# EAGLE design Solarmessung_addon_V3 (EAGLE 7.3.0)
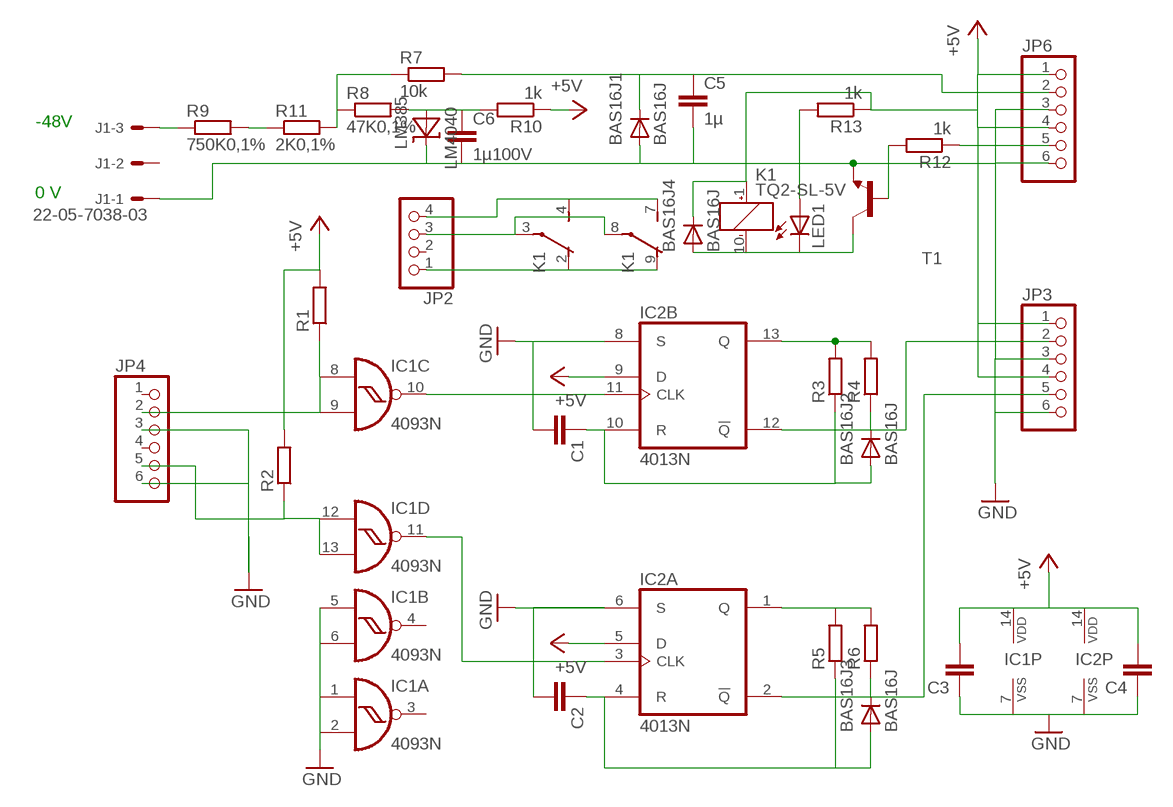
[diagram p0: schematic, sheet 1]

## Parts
BAS16J1  BAS16J  [SOD323-W]
BAS16J2  BAS16J  [SOD323-W]
BAS16J3  BAS16J  [SOD323-W]
BAS16J4  BAS16J  [SOD323-W]
C1  C-EUC1206  [C1206]
C2  C-EUC1206  [C1206]
C3  C-EUC1206  [C1206]
C4  C-EUC1206  [C1206]
C5  1µ  C-EUC0805  [C0805]
C6  1µ100V  C-EUC1206  [C1206]
IC1  4093N  [DIL14]
IC2  4013N  [DIL14]
J1  22-05-7038-03  [7395-03]
JP2  PINHD-1X4  [1X04]
JP3  PINHD-1X6  [1X06]
JP4  PINHD-1X6  [1X06]
JP6  PINHD-1X6  [1X06]
K1  TQ2-SL-5V  [TQ-SL]
LED1  LED3MM  [LED3MM]
LM4040  LM385  [TO-92]
R1  R-EU_R1206  [R1206]
R2  R-EU_R1206  [R1206]
R3  R-EU_R0603  [R0603]
R4  R-EU_R0603  [R0603]
R5  R-EU_R0603  [R0603]
R6  R-EU_R0603  [R0603]
R7  10k  R-EU_M1206  [M1206]
R8  47K0,1%  R-EU_M1206  [M1206]
R9  750K0,1%  R-EU_M1206  [M1206]
R10  1k  R-EU_M1206  [M1206]
R11  2K0,1%  R-EU_M1206  [M1206]
R12  1k  R-EU_R0603  [R0603]
R13  1k  R-EU_R0603  [R0603]
T1  -NPN-SOT23-EBC  [SOT23-EBC]

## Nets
+5V: BAS16J4.C C3.2 C4.2 IC1.14(P:VDD) IC2.5(A:D) IC2.9(B:D) IC2.14(P:VDD) JP3.1 JP3.4 JP6.1 JP6.4 K1.1(_:+) R1.2 R2.2 R10.1 R13.1
GND: BAS16J1.A C1.2 C2.2 C3.1 C4.1 C5.2 C6.2 IC1.1(A:I0) IC1.2(A:I1) IC1.5(B:I0) IC1.6(B:I1) IC1.7(P:VSS) IC2.6(A:S) IC2.7(P:VSS) IC2.8(B:S) J1.1 JP3.3 JP3.6 JP4.3 JP4.6 JP6.3 JP6.6 LM4040.- T1.E
N$1: IC1.8(C:I0) IC1.9(C:I1) JP4.2 R1.1
N$2: IC1.12(D:I0) IC1.13(D:I1) JP4.5 R2.1
N$3: C6.1 LM4040.+ R8.2 R10.2
N$4: IC1.10(C:O) IC2.11(B:CLK)
N$5: BAS16J2.C R4.1
N$6: BAS16J2.A C1.1 IC2.10(B:R) R3.1
N$7: IC2.13(B:Q) R3.2 R4.2
N$8: IC1.11(D:O) IC2.3(A:CLK)
N$9: BAS16J3.C R6.1
N$10: BAS16J3.A C2.1 IC2.4(A:R) R5.1
N$11: IC2.1(A:Q) R5.2 R6.2
N$12: J1.3 R9.1
N$13: R7.1 R8.1 R11.2
N$14: BAS16J1.C C5.1 JP6.2 R7.2
N$15: R9.2 R11.1
N$16: R12.2 T1.B
N$17: JP6.5 R12.1
N$18: BAS16J4.A K1.10(_:-) LED1.K(C) T1.C
N$19: JP2.4 K1.4(1:S) K1.7(2:S)
N$20: JP2.3 K1.3(1:P) K1.8(2:P)
N$21: JP2.1 K1.2(1:O) K1.9(2:O)
N$22: IC2.12(B:!Q) JP3.2
N$23: LED1.A R13.2
N$24: IC2.2(A:!Q) JP3.5
Unconnected: IC1.3(A:O) IC1.4(B:O) J1.2 JP2.2 JP4.1 JP4.4

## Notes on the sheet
- -48V
- 0 V

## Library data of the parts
BAS16J1-BAS16J4 = diode:BAS16J
C1-C6 = rcl:C-EU: CAPACITOR, European symbol
IC1 = 40xx:4093: Quad 2-input NAND schmitt trigger
IC2 = 40xx:4013: Dual D FLIP FLOP, set/reset
J1 = con-molex:22-?-03: CONNECTOR wire to board 2.54 mm (.1 inch) pitch header
JP2 = pinhead:PINHD-1X4: PIN HEADER
JP3 JP4 JP6 = pinhead:PINHD-1X6: PIN HEADER
K1 = relay:TQ2?*: LOW PROFILE 2 FORM C RELAY NAiS Source: http://www.mew-europe.com/.. en_ds_61020_0001.pdf Source: http://www.mew-europe.com/.. en_ds_61020_0004.pdf
LED1 = led:LED: LED
LM4040 = lm385:LM385: LM385
R1-R13 = rcl:R-EU_: RESISTOR, European symbol
T1 = transistor:*-NPN-: NPN Transistror BF959 corrected 2008.03.06

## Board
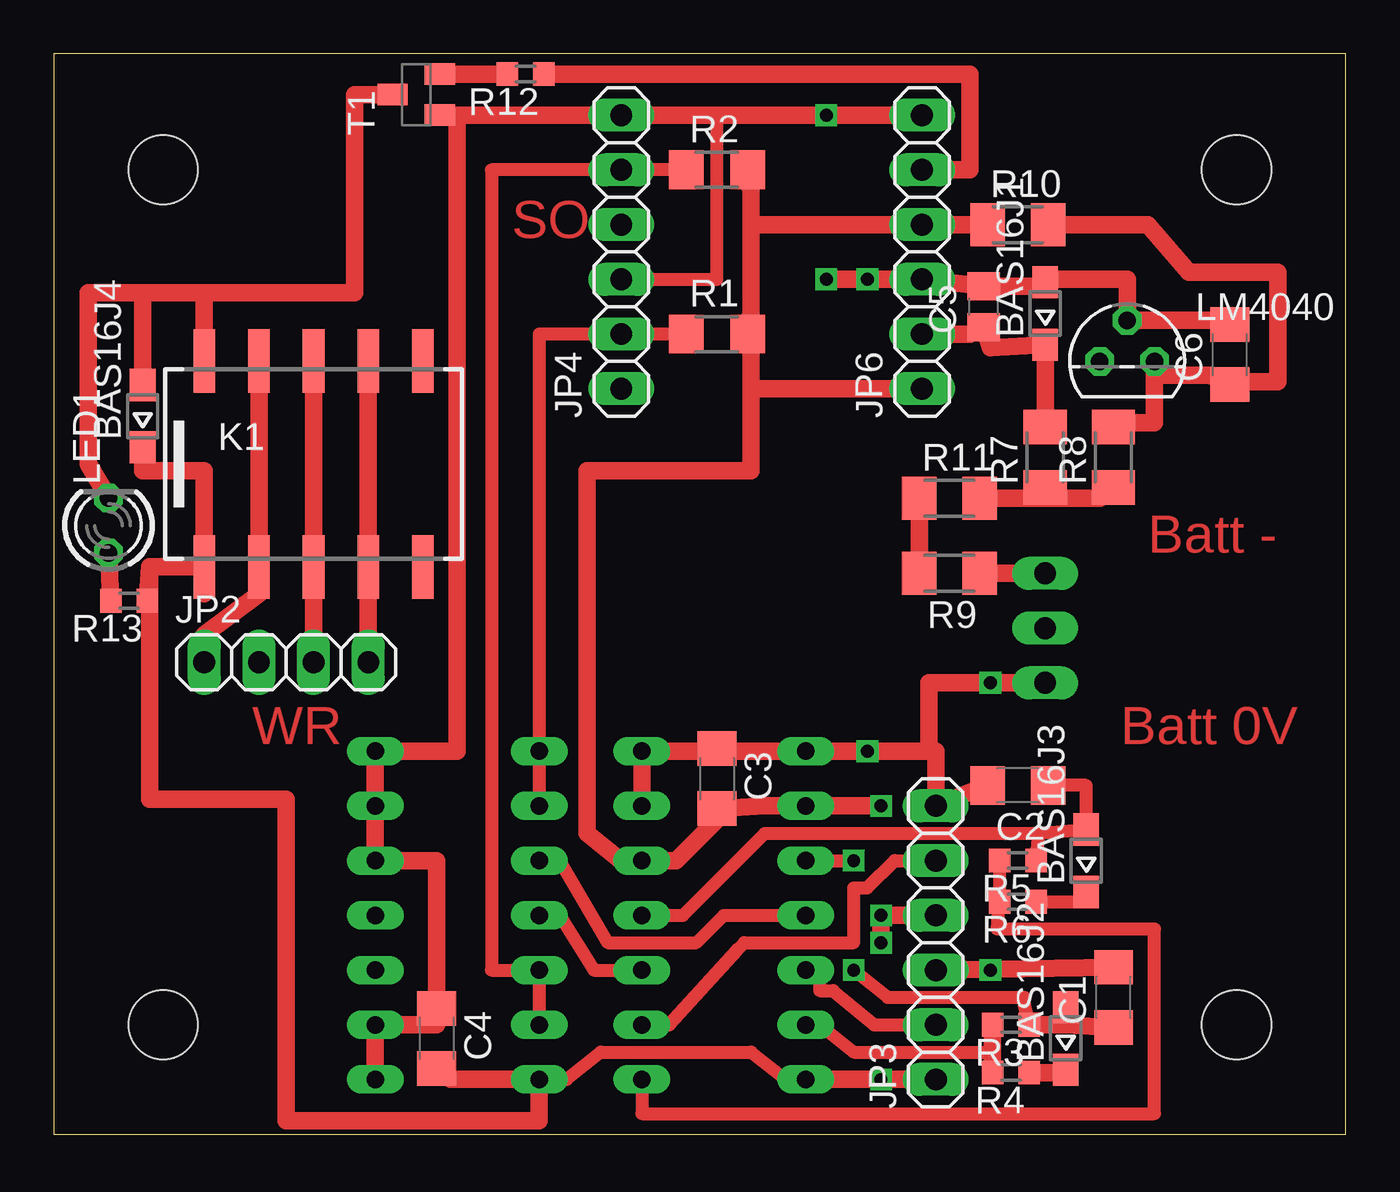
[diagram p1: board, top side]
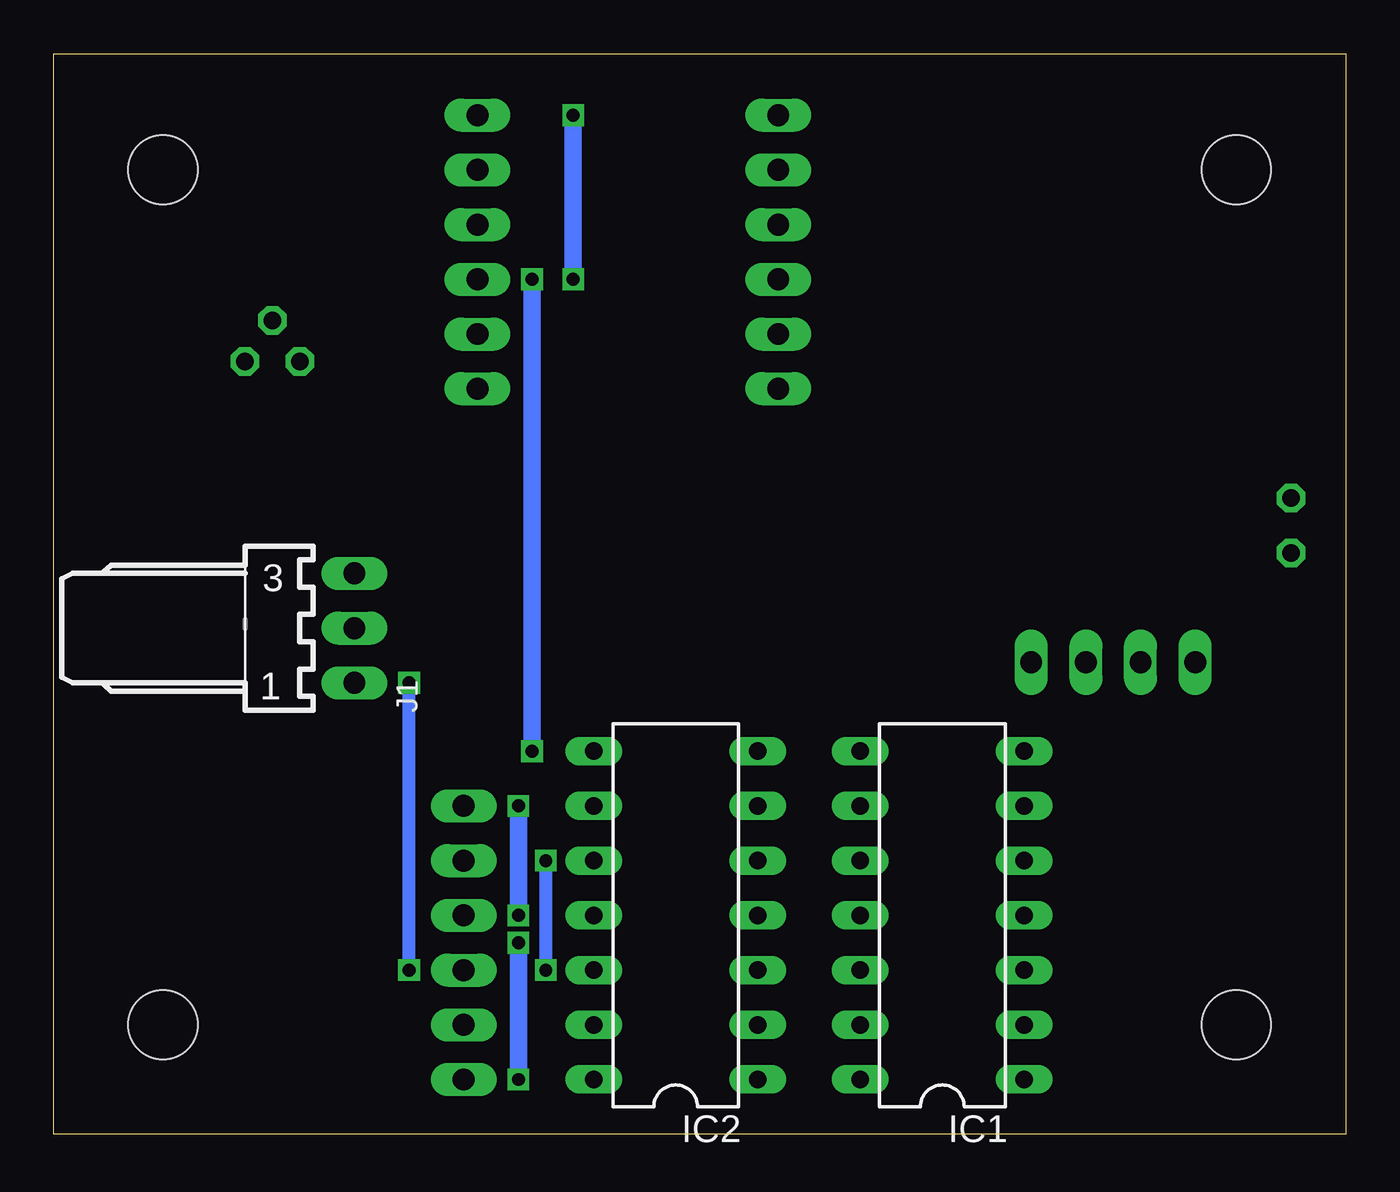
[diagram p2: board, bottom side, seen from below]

Size 59.99 x 50.16 mm. Coordinates in mm from the lower left corner, seen from the top.
Outline: 0,0 59.99,0 59.99,50.16 0,50.16 0,0
Copper layers (1*16): Top 0.035mm / dielectric 1.5mm / Bottom 0.035mm
Design rules "default": minimum track width 10mil, minimum drill 24mil, track to track 8mil, track to pad 8mil, pad to pad 8mil, via to via 8mil, smd to smd 8mil, copper to edge 40mil, drill to drill 8mil, minimum pad ring 10mil, minimum via ring 8mil, stop-mask expansion 4mil, vias tented up to drill 0mil, thermal gap 10mil
Holes 3.2 mm at 5.08,5.08 54.93,5.08 5.08,44.77 54.93,44.77

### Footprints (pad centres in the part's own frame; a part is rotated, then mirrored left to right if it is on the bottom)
SOD323-W = smd 1.5 x 1.2: A 1.45,0; C -1.45,0
C1206 = smd 1.6 x 1.8: 1 -1.4,0; 2 1.4,0
C0805 = smd 1.3 x 1.5: 1 -0.95,0; 2 0.95,0
DIL14 = drill 0.813 long: 1 -7.62,-3.81; 2 -5.08,-3.81; 3 -2.54,-3.81; 4 0,-3.81; 5 2.54,-3.81; 6 5.08,-3.81; 7 7.62,-3.81; 8 7.62,3.81; 9 5.08,3.81; 10 2.54,3.81; 11 0,3.81; 12 -2.54,3.81; 13 -5.08,3.81; 14 -7.62,3.81
7395-03 = drill 1.016 long: 1 2.54,0; 2 0,0; 3 -2.54,0
1X04 = drill 1.016 long: 1 -3.81,0; 2 -1.27,0; 3 1.27,0; 4 3.81,0
1X06 = drill 1.016 long: 1 -6.35,0; 2 -3.81,0; 3 -1.27,0; 4 1.27,0; 5 3.81,0; 6 6.35,0
TQ-SL = smd 1 x 2.94: 1 -5.08,-4.78; 2 -2.54,-4.78; 3 0,-4.78; 4 2.54,-4.78; 5 5.08,-4.78; 6 5.08,4.78; 7 2.54,4.78; 8 0,4.78; 9 -2.54,4.78; 10 -5.08,4.78
LED3MM = drill 0.813 octagon: A -1.27,0; K 1.27,0
TO-92 = drill 0.813 octagon: + 1.27,0; - 0,1.905; NC -1.27,0
R1206 = smd 1.6 x 1.803: 1 -1.422,0; 2 1.422,0
R0603 = smd 1 x 1.1: 1 -0.85,0; 2 0.85,0
M1206 = smd 1.6 x 2: 1 -1.4,0; 2 1.4,0
SOT23-EBC = smd 1 x 1.4: B 0.95,-1.1; C 0,1.1; E -0.95,-1.1

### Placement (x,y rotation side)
BAS16J1  46.04,38.1 90 top
BAS16J2  46.99,4.45 90 top
BAS16J3  47.94,12.7 90 top
BAS16J4  4.13,33.34 90 top
C1  49.21,6.35 90 top
C2  44.77,16.19 180 top
C3  30.8,16.51 270 top
C4  17.78,4.45 270 top
C5  43.18,38.42 90 top
C6  54.61,36.2 90 top
IC1  18.73,10.16 90 bottom
IC2  31.11,10.16 90 bottom
J1  46.04,23.5 270 bottom
JP2  10.79,21.91 0 top
JP3  40.96,8.89 90 top
JP4  26.35,40.96 90 top
JP6  40.32,40.96 90 top
K1  12.06,31.11 0 top
LED1  2.54,28.26 90 top
LM4040  49.85,35.88 0 top
R1  30.8,37.15 0 top
R2  30.8,44.77 0 top
R3  44.45,5.08 180 top
R4  44.45,2.86 180 top
R5  44.77,12.7 180 top
R6  44.77,10.79 180 top
R7  46.04,31.43 90 top
R8  49.21,31.43 90 top
R9  41.59,26.04 180 top
R10  44.77,42.23 0 top
R11  41.59,29.53 0 top
R12  21.91,49.21 180 top
R13  3.49,24.77 180 top
T1  16.83,48.26 90 top

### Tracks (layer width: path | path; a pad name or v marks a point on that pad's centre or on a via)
+5V  (via drill 0.6)
  Top 0.61: IC1.14 23.81,2.54 25.4,3.81 32.38,3.81 33.97,2.54 IC2.14 | 34.29,15.24 IC2.9
  Top 0.813: R10.1 JP6.4 32.38,42.23 | IC2.14 v38.42,2.54 JP3.1 | BAS16J4.C 4.13,30.8 6.99,30.8 6.99,26.35 | 6.99,25.08 K1.1 6.99,26.35 | 4.45,26.35 R13.1 | 6.99,26.35 4.45,26.35 | 4.45,26.35 4.45,15.56 10.79,15.56 10.79,0.64 22.54,0.64 IC1.14 18.41,2.54 C4.2 | v38.42,8.89 v38.42,10.16 JP3.4 | v38.42,15.24 34.29,15.24 33.02,15.24 C3.2 30.8,14.61 28.89,12.7 IC2.5 26.35,12.7 24.77,13.97 24.77,30.8 32.38,30.8 32.38,34.61 | 32.38,42.23 32.38,43.81 R2.2 | 32.38,42.23 32.38,38.1 R1.2 32.38,36.51 32.38,34.61 | JP6.1 32.38,34.61
  Bottom 0.813: v38.42,8.89 v38.42,2.54 | v38.42,10.16 v38.42,15.24
GND  (via drill 0.6)
  Top 0.61: 43.18,16.19 C2.2 | 30.8,47.31 JP4.6 19.05,47.31 | 30.8,47.31 v35.88,47.31 | JP6.3 40.32,39.37 | JP4.3 30.8,39.69 30.8,47.31 | JP3.3 v43.5,7.62
  Top 0.813: C1.2 JP3.3 | T1.E 18.73,47.31 | 18.73,47.31 JP6.6 v35.88,47.31 | IC1.1 IC1.2 17.78,5.08 C4.1 17.78,12.7 IC1.5 IC1.6 IC1.7 18.73,17.78 18.73,47.31 | v35.88,39.69 v37.78,39.69 JP6.3 C5.2 45.4,39.37 BAS16J1.A 46.67,39.69 49.85,39.69 LM4040.- 53.66,37.78 C6.2 | IC2.6 IC2.7 | IC2.7 30.8,17.78 C3.1 31.75,17.78 IC2.8 | IC2.8 v37.78,17.78 40.64,17.78 | 40.64,17.78 40.96,17.78 JP3.6 42.55,15.88 C2.2 | J1.1 v43.5,20.95 40.64,20.95 40.64,17.78 | IC2.7 IC2.8
  Bottom 0.61: v43.5,7.62 v43.5,20.95
  Bottom 0.813: v35.88,47.31 v35.88,39.69 | v37.78,17.78 v37.78,39.69
N$1
  Top 0.61: IC1.9 IC1.8 22.54,37.15 R1.1 JP4.2
N$2
  Top 0.61: IC1.13 IC1.12 20.32,7.62 20.32,44.77 JP4.5 R2.1
N$3
  Top 0.813: LM4040.+ 51.12,35.24 | 51.12,35.24 51.12,33.02 49.85,33.02 R8.2 | 51.12,35.24 53.66,35.24 C6.1 55.24,34.92 56.83,34.92 56.83,40.01 52.7,40.01 50.8,42.23 R10.2
N$4
  Top 0.61: IC1.10 23.5,12.7 25.72,8.89 29.84,8.89 31.11,10.16 IC2.11
N$5
  Top 0.813: R4.1 46.67,2.86 BAS16J2.C
N$6  (via drill 0.6)
  Top 0.61: R3.1 45.09,6.03 45.09,6.35 38.73,6.35 v37.15,7.62 | IC2.10 v37.15,12.7
  Top 0.813: R3.1 46.99,5.08 | 46.99,5.08 47.31,5.08 BAS16J2.A 46.99,5.08 | 46.99,5.08 C1.1
  Bottom 0.61: v37.15,12.7 v37.15,7.62
N$7
  Top 0.61: IC2.13 35.56,5.08 37.15,3.81 43.6,3.81
  Top 0.813: R4.2 43.6,3.81 R3.2
N$8
  Top 0.61: IC1.11 23.5,10.16 25.08,7.62 IC2.3
N$9
  Top 0.61: R6.1 47.62,10.79 BAS16J3.C
N$10
  Top 0.61: 45.72,13.97 BAS16J3.A 47.94,16.19 C2.1 | IC2.4 29.21,10.16 33.02,13.97 45.72,13.97 | 45.72,13.97 R5.1
N$11
  Top 0.61: R5.2 R6.2 43.81,9.53 51.12,9.53 51.12,0.95 27.3,0.95 IC2.1
N$12
  Top 0.813: J1.3 R9.1
N$13
  Top 0.813: R11.2 46.04,29.53 | 46.04,29.53 48.58,29.53 R8.1 | R7.1 46.04,29.53
N$14
  Top 0.813: R7.2 BAS16J1.C 43.5,36.51 C5.1 42.55,37.15 JP6.2
N$15
  Top 0.813: R11.1 R9.2
N$16
  Top 0.813: T1.B R12.2
N$17
  Top 0.813: R12.1 42.55,49.21 42.55,44.77 JP6.5
N$18
  Top 0.813: LED1.K 1.59,31.11 1.59,39.05 4.13,39.05 | 4.13,39.05 6.99,39.05 | 6.99,39.05 K1.10 | BAS16J4.A 4.13,39.05 | T1.C 13.97,48.26 13.97,39.05 6.99,39.05
N$19
  Top 0.813: K1.7 K1.4 JP2.4
N$20
  Top 0.813: K1.8 K1.3 JP2.3
N$21
  Top 0.813: K1.9 K1.2 9.53,25.08 6.99,23.18 JP2.1
N$22
  Top 0.61: JP3.2 39.37,5.08 38.73,5.08 38.1,5.08 36.2,6.67 35.56,6.67 35.56,7.62 IC2.12
N$23
  Top 0.813: LED1.A R13.2
N$24
  Top 0.61: IC2.2 28.57,5.08 31.75,8.57 32.07,8.89 37.15,8.89 37.15,11.43 37.78,11.43 39.05,12.7 JP3.5

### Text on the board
Top: SO | Batt - | WR | Batt 0V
